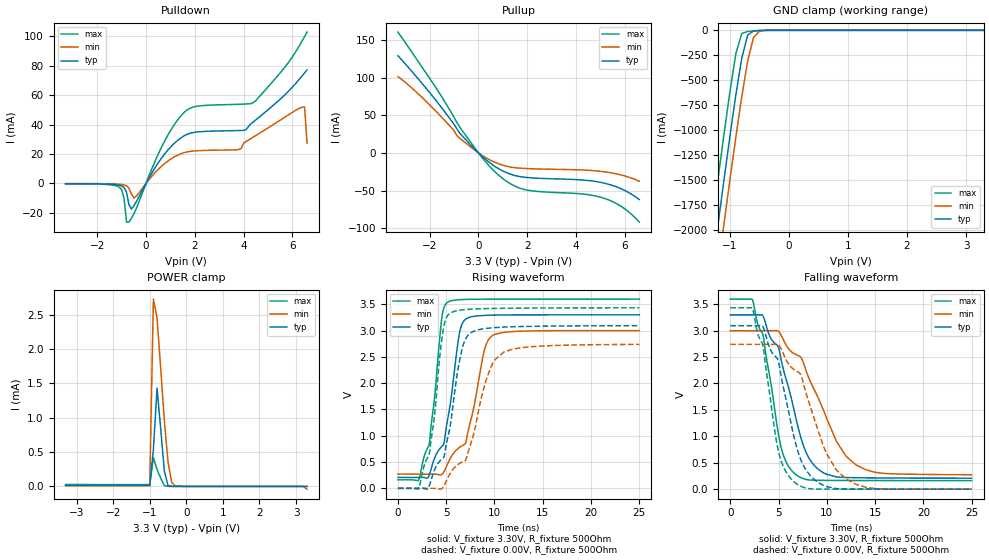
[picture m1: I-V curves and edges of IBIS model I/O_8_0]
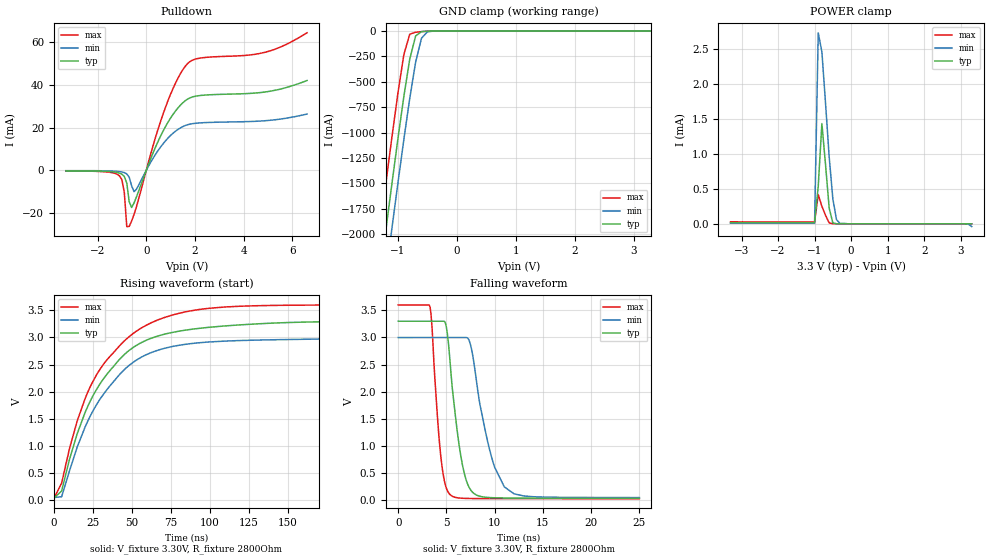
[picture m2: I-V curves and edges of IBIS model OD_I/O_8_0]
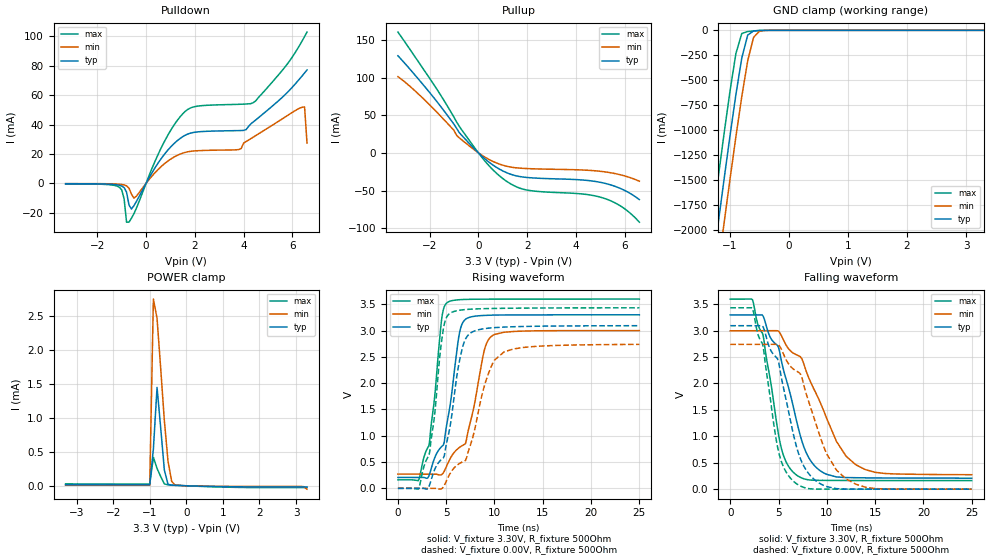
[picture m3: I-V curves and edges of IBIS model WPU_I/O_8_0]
[IBIS Ver]   3.2
[File Name]   lm3s1439_lqfp_v0p1.ibs
[File Rev]   0.1
[Date]   02/19/2010
[Source]   From silicon level SPICE simulations at Texas Instruments
[Notes]   Initial Release of IBIS model
   LM3S1439, Revision A2, 100 LQFP
[Disclaimer] Texas Instruments Confidential - Advance Product Information
   < Software License Agreement >
  Texas Instruments (TI) is supplying this software for use solely and
  exclusively on TI's Stellaris Family of microcontroller products.
  The software is owned by TI and/or its suppliers, and is protected under
  applicable copyright laws.  All rights are reserved.  Any use in violation
  of the foregoing restrictions may subject the user to criminal sanctions
  under applicable laws, as well as to civil liability for the breach of the
  terms and conditions of this license.
  THIS SOFTWARE IS PROVIDED "AS IS".  NO WARRANTIES, WHETHER EXPRESS, IMPLIED
  OR STATUTORY, INCLUDING, BUT NOT LIMITED TO, IMPLIED WARRANTIES OF
  MERCHANTABILITY AND FITNESS FOR A PARTICULAR PURPOSE APPLY TO THIS SOFTWARE.
  LMI SHALL NOT, IN ANY CIRCUMSTANCES, BE LIABLE FOR SPECIAL, INCIDENTAL, OR
  CONSEQUENTIAL DAMAGES, FOR ANY REASON WHATSOEVER.
[Copyright]   Copyright (c) 2010 Texas Instruments.  All rights reserved.
[Component]   LM3S1439 100LQFP
[Manufacturer]  Texas Instruments
[Package]
| 100-pin LQFP
| variable   typ   min   max
R_pkg   125.000m   98.000m   152.000m
L_pkg   7.745nH   6.720nH   8.770nH
C_pkg   0.745pF   0.660pF   0.830pF
[Pin]  signal_name   model_name
   1   ADC0   NC
   2   ADC1   NC
   3   VDDA   POWER
   4   GNDA   GND
   5   ADC2   NC
   6   ADC3   NC
   7   LDO   POWER
   8   VDD   POWER
   9   GND   GND
  10   PD0_PWM0   ProgBuff1
  11   PD1_PWM1   ProgBuff1
  12   PD2_U1Rx   ProgBuff1
  13   PD3_U1Tx   ProgBuff1
  14   VDD25   POWER
  15   GND   GND
  16   PG3   ProgBuff2
  17   PG2   ProgBuff2
  18   PG1   ProgBuff1
  19   PG0   ProgBuff1
  20   VDD   POWER
  21   GND   GND
  22   PC7_PhB0   ProgBuff1
  23   PC6_CCP3   ProgBuff1
  24   PC5_C0o   ProgBuff1
  25   PC4_PhA0   ProgBuff1
  26   PA0_U0Rx   ProgBuff1
  27   PA1_U0Tx   ProgBuff1
  28   PA2_SSI0Clk   ProgBuff1
  29   PA3_SSI0Fss   ProgBuff1
  30   PA4_SSI0Rx   ProgBuff1
  31   PA5_SSI0Tx   ProgBuff1
  32   VDD   POWER
  33   GND   GND
  34   PA6_CCP1   ProgBuff1
  35   PA7_CCP4   ProgBuff1
  36   NC   NC
  37   NC   NC
  38   VDD25   POWER
  39   GND   GND
  40   NC   NC
  41   NC   NC
  42   PF7   ProgBuff2
  43   PF6   ProgBuff2
  44   VDD   POWER
  45   GND   GND
  46   PF5   ProgBuff2
  47   PF0   ProgBuff1
  48   OSC0   NC
  49   OSC1   NC
  50   WAKE   NC
  51   HIB   NC
  52   XOSC0   NC
  53   XOSC1   NC
  54   GND   GND
  55   VBAT   POWER
  56   VDD   POWER
  57   GND   GND
  58   PF4   ProgBuff1
  59   PF3_PWM5   ProgBuff1
  60   PF2_PWM4   ProgBuff1
  61   PF1   ProgBuff1
  62   VDD25   POWER
  63   GND   GND
  64   RST   NC
  65   CMOD0   NC
  66   PB0_CCP0   ProgBuff1
  67   PB1_CCP2   ProgBuff1
  68   VDD   POWER
  69   GND   GND
  70   PB2_I2C0SCL   ProgBuff1
  71   PB3_I2C0SDA   ProgBuff1
  72   PE0_SSI1Clk   ProgBuff1
  73   PE1_SSI1Fss   ProgBuff1
  74   PE2_SSI1Rx   ProgBuff1
  75   PE3_SSI1Tx   ProgBuff1
  76   CMOD1   NC
  77   PC3_TDO_SWO   ProgBuff1
  78   PC2_TDI   ProgBuff1
  79   PC1_TMS_SWDIO   ProgBuff1
  80   PC0_TCK_SWCLK   ProgBuff1
  81   VDD   POWER
  82   GND   GND
  83   PH3   ProgBuff2
  84   PH2   ProgBuff2
  85   PH1_PWM3   ProgBuff2
  86   PH0_PWM2   ProgBuff2
  87   GND   GND
  88   VDD25   POWER
  89   PB7_TRST   ProgBuff1
  90   PB6   ProgBuff1
  91   PB5_CCP5   ProgBuff1
  92   PB4   ProgBuff1
  93   VDD   POWER
  94   GND   GND
  95   PD4   ProgBuff0
  96   PD5   ProgBuff0
  97   GNDA   GND
  98   VDDA   POWER
  99   PD6_Fault   ProgBuff0
 100   PD7_IDX0   ProgBuff0
[Model Selector]   ProgBuff0
I/O_2_0   2 mA buffer without slew rate control
I/O_4_0   4 mA buffer without slew rate control
I/O_8_0   8 mA buffer without slew rate control
I/O_8S_0   8 mA buffer with slew rate control
OD_I/O_2_0   open-drain 2 mA buffer without slew rate control
OD_I/O_4_0   open-drain 4 mA buffer without slew rate control
OD_I/O_8_0   open-drain 8 mA buffer without slew rate control
OD_I/O_8S_0   open-drain 8 mA buffer with slew rate control
WPU_I/O_2_0   weak pullup 2 mA buffer without slew rate control
WPU_I/O_4_0   weak pullup 4 mA buffer without slew rate control
WPU_I/O_8_0   weak pullup 8 mA buffer without slew rate control
WPU_I/O_8S_0   weak pullup 8 mA buffer with slew rate control
WPD_I/O_2_0   weak pulldown 2 mA buffer without slew rate control
WPD_I/O_4_0   weak pulldown 4 mA buffer without slew rate control
WPD_I/O_8_0   weak pulldown 8 mA buffer without slew rate control
WPD_I/O_8S_0   weak pulldown 8 mA buffer with slew rate control
[Model Selector]   ProgBuff1
I/O_2_1   2 mA buffer without slew rate control
I/O_4_1   4 mA buffer without slew rate control
I/O_8_1   8 mA buffer without slew rate control
I/O_8S_1   8 mA buffer with slew rate control
OD_I/O_2_1   open-drain 2 mA buffer without slew rate control
OD_I/O_4_1   open-drain 4 mA buffer without slew rate control
OD_I/O_8_1   open-drain 8 mA buffer without slew rate control
OD_I/O_8S_1   open-drain 8 mA buffer with slew rate control
WPU_I/O_2_1   weak pullup 2 mA buffer without slew rate control
WPU_I/O_4_1   weak pullup 4 mA buffer without slew rate control
WPU_I/O_8_1   weak pullup 8 mA buffer without slew rate control
WPU_I/O_8S_1   weak pullup 8 mA buffer with slew rate control
WPD_I/O_2_1   weak pulldown 2 mA buffer without slew rate control
WPD_I/O_4_1   weak pulldown 4 mA buffer without slew rate control
WPD_I/O_8_1   weak pulldown 8 mA buffer without slew rate control
WPD_I/O_8S_1   weak pulldown 8 mA buffer with slew rate control
[Model Selector]   ProgBuff2
I/O_2_2   2 mA buffer without slew rate control
I/O_4_2   4 mA buffer without slew rate control
I/O_8_2   8 mA buffer without slew rate control
I/O_8S_2   8 mA buffer with slew rate control
OD_I/O_2_2   open-drain 2 mA buffer without slew rate control
OD_I/O_4_2   open-drain 4 mA buffer without slew rate control
OD_I/O_8_2   open-drain 8 mA buffer without slew rate control
OD_I/O_8S_2   open-drain 8 mA buffer with slew rate control
WPU_I/O_2_2   weak pullup 2 mA buffer without slew rate control
WPU_I/O_4_2   weak pullup 4 mA buffer without slew rate control
WPU_I/O_8_2   weak pullup 8 mA buffer without slew rate control
WPU_I/O_8S_2   weak pullup 8 mA buffer with slew rate control
WPD_I/O_2_2   weak pulldown 2 mA buffer without slew rate control
WPD_I/O_4_2   weak pulldown 4 mA buffer without slew rate control
WPD_I/O_8_2   weak pulldown 8 mA buffer without slew rate control
WPD_I/O_8S_2   weak pulldown 8 mA buffer with slew rate control
| Models and submodels in the file (48): I/O_2_0 (I/O), I/O_4_0 (I/O), I/O_8_0 (I/O), I/O_8S_0 (I/O), OD_I/O_2_0 (I/O_open_drain), OD_I/O_4_0 (I/O_open_drain), OD_I/O_8_0 (I/O_open_drain), OD_I/O_8S_0 (I/O_open_drain), WPU_I/O_2_0 (I/O), WPU_I/O_4_0 (I/O), WPU_I/O_8_0 (I/O), WPU_I/O_8S_0 (I/O), WPD_I/O_2_0 (I/O), WPD_I/O_4_0 (I/O), WPD_I/O_8_0 (I/O), WPD_I/O_8S_0 (I/O), I/O_2_1 (I/O), I/O_4_1 (I/O), I/O_8_1 (I/O), I/O_8S_1 (I/O), OD_I/O_2_1 (I/O_open_drain), OD_I/O_4_1 (I/O_open_drain), OD_I/O_8_1 (I/O_open_drain), OD_I/O_8S_1 (I/O_open_drain), WPU_I/O_2_1 (I/O), WPU_I/O_4_1 (I/O), WPU_I/O_8_1 (I/O), WPU_I/O_8S_1 (I/O), WPD_I/O_2_1 (I/O), WPD_I/O_4_1 (I/O), WPD_I/O_8_1 (I/O), WPD_I/O_8S_1 (I/O), I/O_2_2 (I/O), I/O_4_2 (I/O), I/O_8_2 (I/O), I/O_8S_2 (I/O), OD_I/O_2_2 (I/O_open_drain), OD_I/O_4_2 (I/O_open_drain), OD_I/O_8_2 (I/O_open_drain), OD_I/O_8S_2 (I/O_open_drain), WPU_I/O_2_2 (I/O), WPU_I/O_4_2 (I/O), WPU_I/O_8_2 (I/O), WPU_I/O_8S_2 (I/O), WPD_I/O_2_2 (I/O), WPD_I/O_4_2 (I/O), WPD_I/O_8_2 (I/O), WPD_I/O_8S_2 (I/O)
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[Model]   I/O_8_0
Model_type   I/O
Vinl = 1.26
Vinh = 2.04
Vmeas = 1.65
| variable   typ   min   max
C_comp   9.739pF   9.739pF   9.739pF
[Model Spec]
Vinh+   1.91   1.78   2.04
Vinh-   1.90   1.76   2.03
Vinl+   1.40   1.27   1.54
Vinl-   1.39   1.26   1.53
| variable   typ   min   max
[Temperature Range]  25   85   -40
[Voltage Range]   3.3V   3.0V   3.6V
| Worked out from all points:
|   slope of the pulldown table from 0 to 0.495 V, typ, clamps not added: 35.8 ohm
|   slope of the pullup table from 0 to 0.495 V, typ, clamps not added: 35.8 ohm
|   GND clamp passes 1 mA (typ) near -0.48 V on its own axis
|   POWER clamp passes 1 mA (typ) near -0.73 V on its own axis
|   falling waveform, V_fixture 3.30V, R_fixture 500Ohm: 20-80 % time 2.57ns typ, 3.86ns min, 1.79ns max; typ from 3.3 V to 0.208 V
|   rising waveform, V_fixture 3.30V, R_fixture 500Ohm: 20-80 % time 1.44ns typ, 2.05ns min, 1.12ns max; typ from 0.208 V to 3.3 V
|   falling waveform, V_fixture 0.00V, R_fixture 500Ohm: 20-80 % time 2.32ns typ, 3.17ns min, 1.7ns max; typ from 3.09 V to 0 V
|   rising waveform, V_fixture 0.00V, R_fixture 500Ohm: 20-80 % time 1.63ns typ, 2.35ns min, 1.2ns max; typ from 0 V to 3.09 V
[Pulldown]
|  Voltage   I(typ)   I(min)   I(max)
-3.3V     -256.6uA   -145.6uA   -364.5uA
-1.1V     -1.273mA   -587.5uA   -2.567mA
-900mV    -2.885mA   -1.061mA   -10.54mA
-800mV    -5.993mA   -1.67mA    -26.39mA
-700mV    -14.71mA   -3.215mA   -26.33mA
-500mV    -15.26mA   -10mA      -20.66mA
600mV     16.36mA    11.13mA    23.41mA
1.5V      31.68mA    20.52mA    47.2mA
3.8V      35.88mA    22.99mA    53.74mA
4.4V      41.81mA    31.48mA    54.89mA
6.5V      75.06mA    51.95mA    99.78mA
6.6V      77.08mA    27.42mA    102.8mA
[Pullup]
|  Voltage   I(typ)   I(min)   I(max)
-3.3V     128.9mA    101.3mA    160.4mA
-2V       80.13mA    63.77mA    99.04mA
-1V       37.9mA     29.83mA    47.32mA
-700mV    23.81mA    17.7mA     31.28mA
300mV     -8.845mA   -6.303mA   -12.15mA
1V        -23.99mA   -16.37mA   -34.1mA
1.5V      -30.13mA   -19.7mA    -44.22mA
2V        -32.73mA   -20.87mA   -49.46mA
4.3V      -36.12mA   -22.8mA    -54.75mA
5.1V      -39.81mA   -24.88mA   -59.77mA
5.9V      -48.4mA    -29.75mA   -72.06mA
6.6V      -62.06mA   -37.61mA   -92.08mA
[GND Clamp]
|  Voltage   I(typ)   I(min)   I(max)
-3.3V     -11.72A    -12.12A    -11.3A
-1.4V     -2.845A    -3.285A    -2.387A
-1.3V     -2.39A     -2.831A    -1.93A
-1.2V     -1.938A    -2.38A     -1.478A
-1.1V     -1.494A    -1.934A    -1.036A
-1V       -1.059A    -1.496A    -610.6mA
-900mV    -645mA     -1.069A    -232.9mA
-800mV    -277.1mA   -664.4mA   -31.59mA
-700mV    -48.56mA   -306.6mA   -12.09mA
-600mV    -5.558mA   -70.2mA    -6.272mA
-500mV    -1.167mA   -7.88mA    -2.167mA
3.3V      2.282nA    3.101uA    451.3pA
[POWER Clamp]
|  Voltage   I(typ)   I(min)   I(max)
-3.3V     15.18uA    8.315uA    27.48uA
-1V       14.14uA    7.74uA     25.63uA
-900mV    536uA      2.726mA    416.7uA
-800mV    1.43mA     2.454mA    247.6uA
-700mV    840.7uA    1.719mA    119.9uA
-600mV    221.2uA    951.5uA    11.58uA
-500mV    12.35uA    355.6uA    955.3nA
-400mV    305.2nA    58.59uA    44.3nA
-300mV    9.515nA    3.101uA    1.472nA
3.1V      1.302nA    -112.7nA   143.5pA
3.2V      1.207nA    -2.287uA   131.7pA
3.3V      -104.8pA   -40.34uA   119.2pA
[Ramp]
| variable   typ   min   max
dV/dt_f   1.85/2.57n   1.63/3.86n   2.06/1.79n
dV/dt_r   1.86/1.63n   1.64/2.35n   2.06/1.20n
R_load = 500Ohm
[Falling Waveform]
V_fixture = 3.30V
V_fixture_min = 3.00V
V_fixture_max = 3.60V
R_fixture = 500Ohm
|   Time   V(typ)   V(min)   V(max)
0s        3.298V     2.997V     3.597V
2.3ns     3.298V     2.998V     3.585V
3.4ns     3.276V     2.999V     2.915V
5.3ns     2.425V     2.905V     768.3mV
6.8ns     1.342V     2.547V     275.7mV
7.8ns     718.5mV    2.267V     187.4mV
8.9ns     411.5mV    1.807V     167.9mV
11ns      231.5mV    902.7mV    164.8mV
13ns      216.8mV    461.7mV    163.7mV
25ns      208.1mV    273.3mV    162.3mV
[Rising Waveform]
V_fixture = 3.30V
V_fixture_min = 3.00V
V_fixture_max = 3.60V
R_fixture = 500Ohm
|   Time   V(typ)   V(min)   V(max)
0s        207.6mV    270.8mV    162.2mV
2.1ns     207.5mV    270.3mV    146.3mV
3.2ns     232.4mV    270mV      805.7mV
4.5ns     789mV      258.8mV    3.176V
5.1ns     1.262V     447.4mV    3.532V
6.6ns     3.106V     806.1mV    3.588V
7.1ns     3.226V     929.8mV    3.592V
9ns       3.288V     2.662V     3.596V
9.8ns     3.293V     2.906V     3.597V
25ns      3.299V     2.999V     3.598V
[Falling Waveform]
V_fixture = 0.00V
V_fixture_min = 0.00V
V_fixture_max = 0.00V
R_fixture = 500Ohm
|   Time   V(typ)   V(min)   V(max)
0s        3.093V     2.74V      3.433V
2.3ns     3.093V     2.74V      3.421V
3.4ns     3.071V     2.741V     2.706V
5ns       2.413V     2.729V     711.4mV
6.8ns     844mV      2.241V     111.1mV
7.4ns     518mV      2.122V     48.36mV
8.7ns     183.7mV    1.335V     2.419mV
10ns      48.12mV    663.5mV    981.6uV
12ns      1.875mV    192.7mV    82.37uV
25ns      33.93uV    47.46uV    17.48uV
[Rising Waveform]
V_fixture = 0.00V
V_fixture_min = 0.00V
V_fixture_max = 0.00V
R_fixture = 500Ohm
|   Time   V(typ)   V(min)   V(max)
0s        193.7uV    2.804mV    103.6uV
2.1ns     125.6uV    574.1uV    -15.02mV
3.2ns     26.93mV    301.2uV    615.4mV
4.7ns     577.9mV    27.17mV    3.028V
5.4ns     1.177V     280.6mV    3.328V
6.3ns     2.353V     463.7mV    3.383V
7ns       2.839V     531.8mV    3.399V
9.3ns     3.044V     2.145V     3.418V
11ns      3.066V     2.596V     3.423V
25ns      3.092V     2.737V     3.432V
[Model]   OD_I/O_8_0
Model_type   I/O_open_drain
Polarity   Inverting
Vinl = 1.26
Vinh = 2.04
Vmeas = 1.65
Rref = 2800
Vref = 3.3
| variable   typ   min   max
C_comp   9.739pF   9.739pF   9.739pF
[Model Spec]
Vinh+   1.91   1.78   2.04
Vinh-   1.90   1.76   2.03
Vinl+   1.40   1.27   1.54
Vinl-   1.39   1.26   1.53
| variable   typ   min   max
[Temperature Range]  25   85   -40
[Voltage Range]   3.3V   3.0V   3.6V
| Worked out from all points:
|   slope of the pulldown table from 0 to 0.495 V, typ, clamps not added: 35.8 ohm
|   GND clamp passes 1 mA (typ) near -0.48 V on its own axis
|   POWER clamp passes 1 mA (typ) near -0.73 V on its own axis
|   falling waveform, V_fixture 3.30V, R_fixture 2800Ohm: 20-80 % time 1.29ns typ, 1.99ns min, 858ps max; typ from 3.3 V to 0.038 V
|   rising waveform, V_fixture 3.30V, R_fixture 2800Ohm: 20-80 % time 34.3ns typ, 34ns min, 35.1ns max; typ from 0.038 V to 3.3 V
[Pulldown]
|  Voltage   I(typ)   I(min)   I(max)
-3.3V     -256.6uA   -145.6uA   -364.5uA
-1.1V     -1.273mA   -587.5uA   -2.567mA
-900mV    -2.885mA   -1.061mA   -10.54mA
-800mV    -5.993mA   -1.67mA    -26.39mA
-700mV    -14.71mA   -3.215mA   -26.33mA
-600mV    -17.43mA   -7.321mA   -23.73mA
-500mV    -15.26mA   -10mA      -20.66mA
700mV     18.62mA    12.61mA    26.75mA
1.2V      27.84mA    18.36mA    40.91mA
1.7V      33.44mA    21.41mA    50.13mA
4.9V      36.8mA     23.3mA     55.47mA
6.6V      42.15mA    26.42mA    64.53mA
[GND Clamp]
|  Voltage   I(typ)   I(min)   I(max)
-3.3V     -11.72A    -12.12A    -11.3A
-1.4V     -2.845A    -3.285A    -2.387A
-1.3V     -2.39A     -2.831A    -1.93A
-1.2V     -1.938A    -2.38A     -1.478A
-1.1V     -1.494A    -1.934A    -1.036A
-1V       -1.059A    -1.496A    -610.6mA
-900mV    -645mA     -1.069A    -232.9mA
-800mV    -277.1mA   -664.4mA   -31.59mA
-700mV    -48.56mA   -306.6mA   -12.09mA
-600mV    -5.558mA   -70.2mA    -6.272mA
-500mV    -1.167mA   -7.88mA    -2.167mA
3.3V      2.282nA    3.101uA    451.3pA
[POWER Clamp]
|  Voltage   I(typ)   I(min)   I(max)
-3.3V     15.18uA    8.315uA    27.48uA
-1V       14.14uA    7.74uA     25.63uA
-900mV    536uA      2.726mA    416.7uA
-800mV    1.43mA     2.454mA    247.6uA
-700mV    840.7uA    1.719mA    119.9uA
-600mV    221.2uA    951.5uA    11.58uA
-500mV    12.35uA    355.6uA    955.3nA
-400mV    305.2nA    58.59uA    44.3nA
-300mV    9.515nA    3.101uA    1.472nA
3.1V      1.302nA    -112.7nA   143.5pA
3.2V      1.207nA    -2.287uA   131.7pA
3.3V      -104.8pA   -40.34uA   119.2pA
[Ramp]
| variable   typ   min   max
dV/dt_f   1.96/1.29n   1.77/1.99n   2.14/0.86n
dV/dt_r   1.96/34.31n   1.77/33.98n   2.14/35.07n
R_load = 2800Ohm
[Falling Waveform]
V_fixture = 3.30V
V_fixture_min = 3.00V
V_fixture_max = 3.60V
R_fixture = 2800Ohm
|   Time   V(typ)   V(min)   V(max)
0s        3.3V       2.999V     3.6V
3.3ns     3.3V       2.999V     3.564V
4.4ns     3.3V       2.999V     837mV
5ns       3.185V     2.999V     218.4mV
5.4ns     2.495V     2.999V     100.8mV
6.6ns     707.8mV    2.999V     38.14mV
7.9ns     119.4mV    2.471V     32.01mV
9.4ns     51.42mV    986.7mV    30.54mV
11ns      42.38mV    246.7mV    30.11mV
25ns      37.9mV     50.24mV    29.43mV
[Rising Waveform]
V_fixture = 3.30V
V_fixture_min = 3.00V
V_fixture_max = 3.60V
R_fixture = 2800Ohm
|   Time   V(typ)   V(min)   V(max)
0s        38mV       50.64mV    29.45mV
5ns       171.3mV    65.99mV    317.2mV
10ns      749.4mV    538.2mV    948.2mV
15ns      1.228V     982.3mV    1.463V
26ns      1.974V     1.694V     2.24V
44ns      2.652V     2.374V     2.902V
61ns      2.969V     2.704V     3.25V
83ns      3.129V     2.868V     3.463V
110ns     3.213V     2.933V     3.562V
250ns     3.298V     2.994V     3.599V
[Model]   WPU_I/O_8_0
Model_type   I/O
Vinl = 1.26
Vinh = 2.04
Vmeas = 1.65
| variable   typ   min   max
C_comp   9.739pF   9.739pF   9.739pF
[Model Spec]
Vinh+   1.91   1.78   2.04
Vinh-   1.90   1.76   2.03
Vinl+   1.40   1.27   1.54
Vinl-   1.39   1.26   1.53
| variable   typ   min   max
[Temperature Range]  25   85   -40
[Voltage Range]   3.3V   3.0V   3.6V
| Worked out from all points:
|   slope of the pulldown table from 0 to 0.495 V, typ, clamps not added: 35.8 ohm
|   slope of the pullup table from 0 to 0.495 V, typ, clamps not added: 35.8 ohm
|   GND clamp passes 1 mA (typ) near -0.48 V on its own axis
|   POWER clamp passes 1 mA (typ) near -0.73 V on its own axis
|   falling waveform, V_fixture 3.30V, R_fixture 500Ohm: 20-80 % time 2.57ns typ, 3.86ns min, 1.79ns max; typ from 3.3 V to 0.208 V
|   rising waveform, V_fixture 3.30V, R_fixture 500Ohm: 20-80 % time 1.44ns typ, 2.05ns min, 1.12ns max; typ from 0.208 V to 3.3 V
|   falling waveform, V_fixture 0.00V, R_fixture 500Ohm: 20-80 % time 2.32ns typ, 3.17ns min, 1.7ns max; typ from 3.09 V to 0 V
|   rising waveform, V_fixture 0.00V, R_fixture 500Ohm: 20-80 % time 1.63ns typ, 2.35ns min, 1.2ns max; typ from 0 V to 3.09 V
[Pulldown]
|  Voltage   I(typ)   I(min)   I(max)
-3.3V     -256.4uA   -145.5uA   -364.3uA
-1.1V     -1.272mA   -586.9uA   -2.565mA
-900mV    -2.884mA   -1.06mA    -10.53mA
-800mV    -5.991mA   -1.669mA   -26.38mA
-700mV    -14.71mA   -3.213mA   -26.31mA
-500mV    -15.24mA   -9.997mA   -20.64mA
600mV     16.38mA    11.14mA    23.43mA
1.5V      31.7mA     20.53mA    47.23mA
3.8V      35.88mA    22.99mA    53.74mA
4.4V      41.81mA    31.48mA    54.88mA
6.5V      75.06mA    51.95mA    99.78mA
6.6V      77.08mA    27.42mA    102.8mA
[Pullup]
|  Voltage   I(typ)   I(min)   I(max)
-3.3V     128.9mA    101.3mA    160.4mA
-2V       80.13mA    63.77mA    99.04mA
-1V       37.9mA     29.83mA    47.32mA
-700mV    23.8mA     17.69mA    31.27mA
300mV     -8.84mA    -6.3mA     -12.15mA
1V        -23.98mA   -16.37mA   -34.08mA
1.5V      -30.12mA   -19.69mA   -44.19mA
2V        -32.71mA   -20.86mA   -49.43mA
4.3V      -36.12mA   -22.8mA    -54.73mA
5.1V      -39.81mA   -24.88mA   -59.77mA
5.9V      -48.4mA    -29.75mA   -72.06mA
6.6V      -62.06mA   -37.61mA   -92.08mA
[GND Clamp]
|  Voltage   I(typ)   I(min)   I(max)
-3.3V     -11.72A    -12.12A    -11.3A
-1.4V     -2.845A    -3.285A    -2.387A
-1.3V     -2.39A     -2.831A    -1.93A
-1.2V     -1.938A    -2.38A     -1.478A
-1.1V     -1.494A    -1.934A    -1.036A
-1V       -1.059A    -1.496A    -610.6mA
-900mV    -645mA     -1.069A    -232.9mA
-800mV    -277.1mA   -664.4mA   -31.6mA
-700mV    -48.56mA   -306.6mA   -12.11mA
-600mV    -5.565mA   -70.2mA    -6.295mA
-500mV    -1.181mA   -7.883mA   -2.191mA
3.3V      2.282nA    6.919uA    -6.845uA
[POWER Clamp]
|  Voltage   I(typ)   I(min)   I(max)
-3.3V     15.18uA    8.315uA    27.48uA
-1V       14.14uA    7.74uA     25.63uA
-900mV    539.2uA    2.746mA    419.4uA
-800mV    1.446mA    2.463mA    255uA
-700mV    851uA      1.726mA    135.8uA
-600mV    231.3uA    957.3uA    27.23uA
-500mV    21.69uA    361.2uA    14.14uA
-400mV    7.764uA    63.51uA    10.49uA
-300mV    5.5uA      6.919uA    7.727uA
3.1V      -16.64uA   -9.947uA   -27.43uA
3.2V      -16.65uA   -12.11uA   -27.44uA
3.3V      -16.65uA   -49.87uA   -27.45uA
[Ramp]
| variable   typ   min   max
dV/dt_f   1.85/2.57n   1.63/3.86n   2.06/1.79n
dV/dt_r   1.86/1.63n   1.64/2.35n   2.06/1.20n
R_load = 500Ohm
[Falling Waveform]
V_fixture = 3.30V
V_fixture_min = 3.00V
V_fixture_max = 3.60V
R_fixture = 500Ohm
|   Time   V(typ)   V(min)   V(max)
0s        3.298V     2.997V     3.597V
2.3ns     3.298V     2.998V     3.585V
3.4ns     3.276V     2.999V     2.915V
5.3ns     2.425V     2.905V     768.3mV
6.8ns     1.342V     2.547V     275.7mV
7.8ns     718.5mV    2.267V     187.4mV
8.9ns     411.5mV    1.807V     167.9mV
11ns      231.5mV    902.7mV    164.8mV
13ns      216.8mV    461.7mV    163.7mV
25ns      208.1mV    273.3mV    162.3mV
[Rising Waveform]
V_fixture = 3.30V
V_fixture_min = 3.00V
V_fixture_max = 3.60V
R_fixture = 500Ohm
|   Time   V(typ)   V(min)   V(max)
0s        207.6mV    270.8mV    162.2mV
2.1ns     207.5mV    270.3mV    146.3mV
3.2ns     232.4mV    270mV      805.7mV
4.5ns     789mV      258.8mV    3.176V
5.1ns     1.262V     447.4mV    3.532V
6.6ns     3.106V     806.1mV    3.588V
7.1ns     3.226V     929.8mV    3.592V
9ns       3.288V     2.662V     3.596V
9.8ns     3.293V     2.906V     3.597V
25ns      3.299V     2.999V     3.598V
[Falling Waveform]
V_fixture = 0.00V
V_fixture_min = 0.00V
V_fixture_max = 0.00V
R_fixture = 500Ohm
|   Time   V(typ)   V(min)   V(max)
0s        3.093V     2.74V      3.433V
2.3ns     3.093V     2.74V      3.421V
3.4ns     3.071V     2.741V     2.706V
5ns       2.413V     2.729V     711.4mV
6.8ns     844mV      2.241V     111.1mV
7.4ns     518mV      2.122V     48.36mV
8.7ns     183.7mV    1.335V     2.419mV
10ns      48.12mV    663.5mV    981.6uV
12ns      1.875mV    192.7mV    82.37uV
25ns      33.93uV    47.46uV    17.48uV
[Rising Waveform]
V_fixture = 0.00V
V_fixture_min = 0.00V
V_fixture_max = 0.00V
R_fixture = 500Ohm
|   Time   V(typ)   V(min)   V(max)
0s        193.9uV    2.805mV    104.1uV
2.1ns     125.6uV    574.4uV    -15.02mV
3.2ns     26.93mV    301.2uV    615.4mV
4.7ns     577.9mV    27.17mV    3.028V
5.4ns     1.177V     280.6mV    3.328V
6.3ns     2.353V     463.7mV    3.383V
7ns       2.839V     531.8mV    3.399V
9.3ns     3.044V     2.145V     3.418V
11ns      3.066V     2.596V     3.423V
25ns      3.092V     2.737V     3.432V
